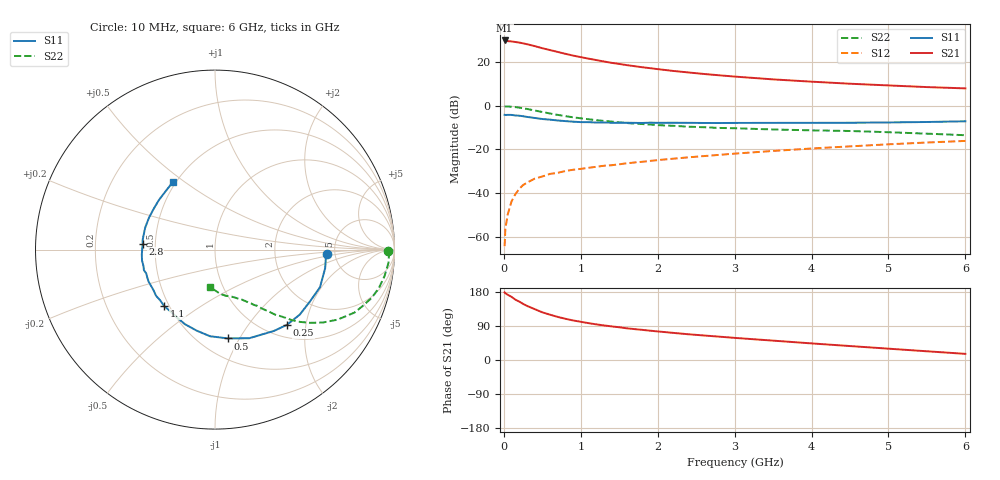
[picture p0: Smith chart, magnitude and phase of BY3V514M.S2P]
! SIEMENS Small Signal Semiconductors
! BFY420
! Si NPN RF SIEGET Grounded Emitter Transistor in MICRO-X
! VCE = 3.5 V  IC = 14 mA
! Common Emitter S-Parameters:  October  1996
# GHz  S  MA  R  50
!  f  S11  S21  S12  S22
! GHz  MAG  ANG  MAG  ANG  MAG  ANG  MAG  ANG
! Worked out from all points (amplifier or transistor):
!   36 points, 10 MHz to 6 GHz, reference 50 ohm
!   highest |S21| = 30.1 dB at 10 MHz (marker M1)
!   |S21| within 3 dB of that: start of sweep to 443 MHz
!   unconditionally stable (mu >= 1): start of sweep to 12.76 MHz; 2.293 GHz to end of sweep
!   at 250 MHz: K = 0.26, MSG = 32.6 dB, |S12| = -36.4 dB
!   at 1.4 GHz: K = 0.84, MSG = 23.5 dB, |S12| = -27.3 dB
!   at 6 GHz: K = 1.08, MAG = 10.4 dB, |S12| = -16.1 dB
!   S11 on the Smith chart (normalised r, x): 10 MHz: 4.30, -0.32; 250 MHz: 1.24, -1.57; 500 MHz: 0.68, -0.89; 1.1 GHz: 0.47, -0.36; 2.8 GHz: 0.42, +0.03; 6 GHz: 0.48, +0.45
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0.01  0.6244 -2.1  31.9 178.5  0.0006 66.0  0.9664 -0.6
0.02  0.6194 -3.9  31.55 176.1  0.0015 61.8  0.9699 -1.5
0.1  0.6214 -19.7  30.29 166.6  0.0064 78.1  0.9561 -8.9
0.15  0.6033 -28.4  29.39 159.3  0.0094 72.5  0.9377 -13.2
0.2  0.5952 -37.5  28.51 154.2  0.0124 73.5  0.9136 -17.1
0.25  0.58 -46.3  27.38 148.1  0.0152 68.8  0.8809 -20.9
0.3  0.5595 -54.1  26.18 142.9  0.0172 67.2  0.8527 -24.3
0.4  0.5294 -68.9  23.7 134.3  0.0213 63.0  0.7859 -29.8
0.5  0.4999 -81.8  21.18 125.8  0.0239 59.4  0.7247 -34.1
0.6  0.4835 -93.3  19.18 119.6  0.0275 57.8  0.6702 -37.5
0.7  0.463 -102.7  17.41 113.7  0.029 56.8  0.623 -40.3
0.8  0.448 -112.0  15.73 108.8  0.032 54.9  0.5822 -42.5
0.9  0.4346 -118.5  14.33 104.4  0.0341 54.1  0.5476 -44.0
1.1  0.4233 -132.1  12.21 97.3  0.0379 55.1  0.4943 -47.2
1.3  0.4172 -142.0  10.5 91.3  0.0422 54.2  0.4523 -49.3
1.6  0.4109 -154.3  8.642 83.6  0.0482 54.2  0.4047 -52.3
2.2  0.411 -171.6  6.365 71.6  0.0613 53.8  0.3492 -57.6
2.8  0.4047 175.5  5.051 61.6  0.0751 51.6  0.3121 -62.4
3.5  0.4078 162.5  4.07 51.1  0.0923 48.3  0.2878 -67.8
4.5  0.4104 146.1  3.235 36.8  0.1177 41.6  0.2655 -76.4
5.5  0.4272 129.4  2.708 23.0  0.1444 33.3  0.2305 -88.8
6  0.4436 122.0  2.528 16.2  0.157 28.8  0.2123 -97.0
